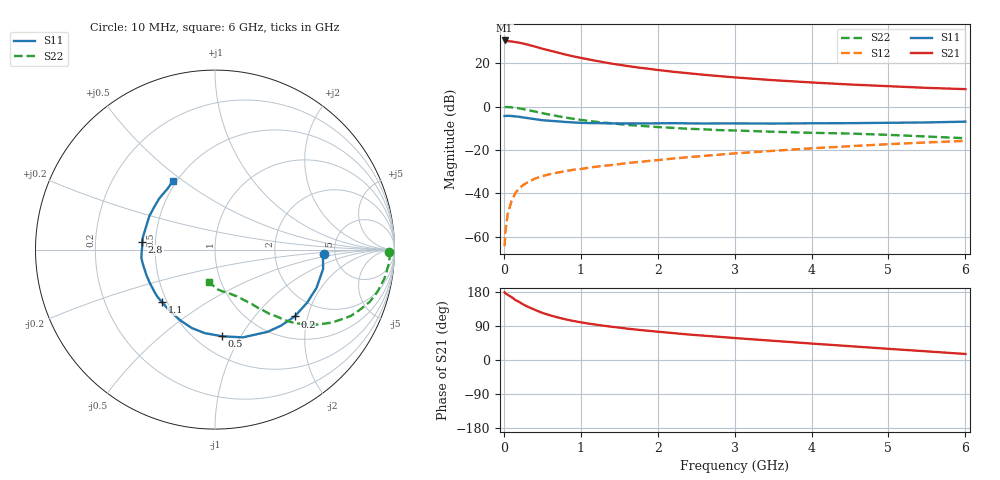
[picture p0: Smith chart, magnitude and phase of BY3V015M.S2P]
! SIEMENS Small Signal Semiconductors
! BFY420
! Si NPN RF SIEGET Grounded Emitter Transistor in MICRO-X
! VCE = 3 V  IC = 15 mA
! Common Emitter S-Parameters:  October  1996
# GHz  S  MA  R  50
!  f  S11  S21  S12  S22
! GHz  MAG  ANG  MAG  ANG  MAG  ANG  MAG  ANG
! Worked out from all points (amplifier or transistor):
!   36 points, 10 MHz to 6 GHz, reference 50 ohm
!   highest |S21| = 30.5 dB at 10 MHz (marker M1)
!   |S21| within 3 dB of that: start of sweep to 422.3 MHz
!   unconditionally stable (mu >= 1): start of sweep to 11.17 MHz; 2.235 GHz to end of sweep
!   at 250 MHz: K = 0.25, MSG = 32.7 dB, |S12| = -36.2 dB
!   at 1.4 GHz: K = 0.85, MSG = 23.4 dB, |S12| = -27.0 dB
!   at 6 GHz: K = 1.08, MAG = 10.3 dB, |S12| = -15.8 dB
!   S11 on the Smith chart (normalised r, x): 10 MHz: 4.09, -0.32; 200 MHz: 1.48, -1.66; 500 MHz: 0.66, -0.83; 1.1 GHz: 0.47, -0.33; 2.8 GHz: 0.42, +0.04; 6 GHz: 0.48, +0.46
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0.01  0.6093 -2.3  33.47 178.7  0.0006 73.3  0.969 -0.7
0.02  0.6033 -4.2  33.06 175.9  0.0013 70.7  0.9744 -1.6
0.1  0.6043 -20.7  31.74 166.0  0.0066 81.7  0.9576 -9.7
0.15  0.5922 -30.0  30.68 158.5  0.0101 74.0  0.9359 -14.4
0.2  0.5796 -40.0  29.73 153.1  0.0129 73.3  0.9102 -18.6
0.25  0.5608 -49.1  28.45 146.9  0.0154 69.6  0.8736 -22.6
0.3  0.5441 -57.3  27.06 141.6  0.0175 67.5  0.8414 -26.1
0.4  0.5131 -72.4  24.33 132.8  0.0216 62.6  0.7693 -31.9
0.5  0.4843 -85.4  21.61 124.3  0.0248 60.0  0.7044 -36.4
0.6  0.469 -96.9  19.5 118.0  0.0276 57.5  0.6475 -40.0
0.7  0.4558 -106.4  17.6 112.4  0.0299 57.3  0.5996 -42.9
0.8  0.4402 -115.2  15.84 107.4  0.0323 55.1  0.5567 -45.1
0.9  0.4298 -121.8  14.43 103.2  0.0347 54.7  0.522 -46.6
1.1  0.4158 -135.5  12.27 96.2  0.0387 55.0  0.4672 -49.8
1.3  0.4118 -144.6  10.52 90.4  0.043 54.5  0.4252 -51.9
1.6  0.4071 -156.9  8.633 82.8  0.0495 54.9  0.378 -55.1
2.2  0.4129 -173.4  6.348 71.0  0.0631 53.7  0.3223 -60.4
2.8  0.4078 174.0  5.036 61.1  0.0776 51.6  0.2856 -65.2
3.5  0.4048 161.0  4.058 50.7  0.0951 47.9  0.2618 -70.5
4.5  0.4135 145.1  3.224 36.5  0.1215 40.8  0.2383 -79.2
5.5  0.4295 128.3  2.696 22.8  0.1485 32.4  0.203 -92.3
6  0.4481 121.4  2.52 15.9  0.1615 27.9  0.1857 -100.9
